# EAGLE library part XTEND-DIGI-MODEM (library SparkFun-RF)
Digi XTend 900 1W RF Transceiver The XTend Modem packs a ton of RF punch into a small, low-power, easy-to-use, and reliable module. Outdoors, with line-of-sight, this module can communicate at up to 40 miles; indoors it can still do up to 3000ft. The module transfers a standard asynchronous serial data stream, operates within the ISM 900MHz frequency band and sustains up to 115.2kbps data throughput. The module comes with an attached RPSMA antenna connector. SparkFun Products XTend 900 1W RPSMA - 40 Mile Range (WRL-09411)
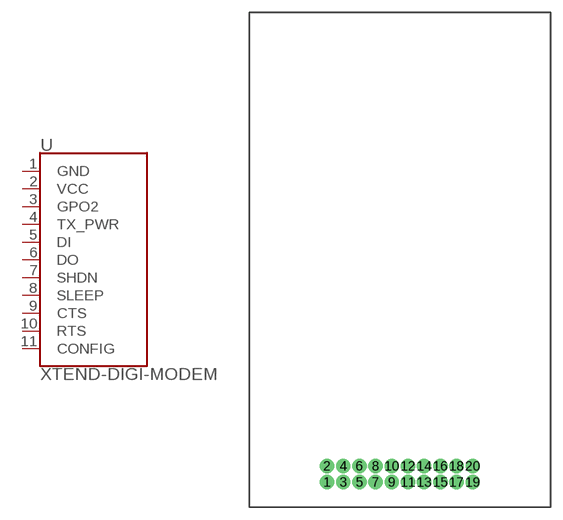
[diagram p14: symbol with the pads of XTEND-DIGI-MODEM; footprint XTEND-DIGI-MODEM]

Designator prefix -

## XTEND-DIGI-MODEM (SF_ID: WRL-09411)  [XTEND-DIGI-MODEM]
1  GND
2  VCC
3  GPO2
4  TX_PWR
5  DI
6  DO
7  SHDN
8  SLEEP
9  CTS
10  RTS
11  CONFIG

## Footprint XTEND-DIGI-MODEM (pad centres in mm)
Digi XTend 900 1W RF Module Module dimensions: 6.05 x 3.65 x 0.51 cm Package for the Xtend Digi Modem 40 mile range. Dimensional Drawing SparkFun Product Link
drill 1.016 pad 1.778: 1 -9,-27.5; 2 -9,-25.5; 3 -7,-27.5; 4 -7,-25.5; 5 -5,-27.5; 6 -5,-25.5; 7 -3,-27.5; 8 -3,-25.5; 9 -1,-27.5; 10 -1,-25.5; 11 1,-27.5; 12 1,-25.5; 13 3,-27.5; 14 3,-25.5; 15 5,-27.5; 16 5,-25.5; 17 7,-27.5; 18 7,-25.5; 19 9,-27.5; 20 9,-25.5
